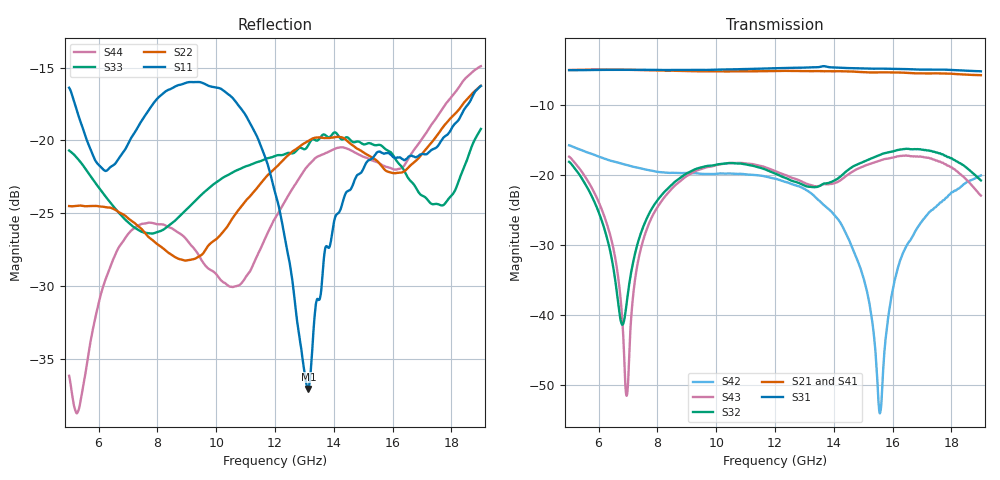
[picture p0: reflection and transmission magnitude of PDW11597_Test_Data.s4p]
!The following data was pulled from an Agilent PNA
!This sNp file was generated from the data in the RF Test software
!NOTE:  Smoothing/Math/Corrections applied on any given trace ARE included in the data saved here
# MHz S dB R 50
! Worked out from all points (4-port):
!   3201 points, 5 GHz to 19 GHz, reference 50 ohm
!   strongest paths, dB at 5 GHz, 8.5 GHz, 12 GHz, 15.5 GHz, 19 GHz:
!     S31: -5.1, -5.0, -4.8, -4.8, -5.2
!     S21: -5.0, -5.1, -5.2, -5.4, -5.8
!     S41: -5.0, -5.1, -5.2, -5.4, -5.8
!     S32: -18.1, -21.4, -19.8, -17.3, -20.8
!     S43: -17.4, -21.9, -19.4, -18.1, -23.0
!     S42: -15.8, -19.7, -20.5, -51.1, -20.1
!   lowest |S11| = -37.1 dB at 13.13 GHz (marker M1), VSWR 1.03, Z = 51.4 + j0.41 ohm
!   |S11| at or under -10 dB: start of sweep to end of sweep
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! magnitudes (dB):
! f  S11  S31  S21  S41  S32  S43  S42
! 5 GHz  -16.4  -5.1  -5.0  -5.0  -18.1  -17.4  -15.8
! 6.956 GHz  -20.4  -5.0  -5.0  -5.0  -38.4  -51.6  -18.6
! 8.452 GHz  -16.5  -5.0  -5.1  -5.1  -21.6  -22.2  -19.7
! 13.13 GHz  -37.1  -4.7  -5.2  -5.2  -21.7  -21.4  -22.4
! 15.57 GHz  -20.8  -4.8  -5.4  -5.4  -17.1  -18.0  -54.0
! 16.38 GHz  -21.3  -4.9  -5.4  -5.4  -16.3  -17.3  -30.9
! 19 GHz  -16.3  -5.2  -5.8  -5.8  -20.8  -23.0  -20.1
